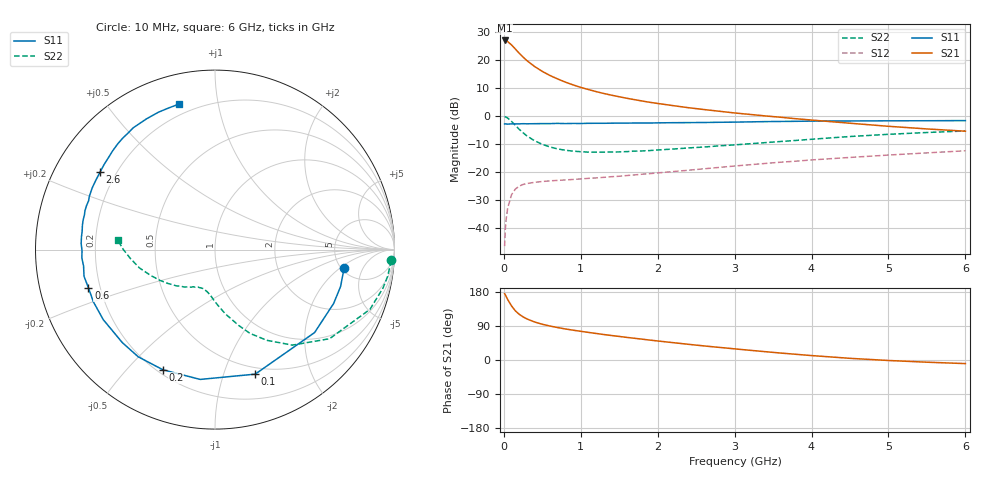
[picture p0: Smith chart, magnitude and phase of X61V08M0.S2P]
! SIEMENS Small Signal Semiconductors
! BFP193W
! Si NPN RF Bipolar Junction Transistor in SOT343
! VCE = 1 V  IC = 8 mA
! Common Emitter S-Parameters:  April 1994
# GHz  S  MA  R  50
!  f  S11  S21  S12  S22
! GHz  MAG  ANG  MAG  ANG  MAG  ANG  MAG  ANG
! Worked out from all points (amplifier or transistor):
!   40 points, 10 MHz to 6 GHz, reference 50 ohm
!   highest |S21| = 27.1 dB at 10 MHz (marker M1)
!   |S21| within 3 dB of that: start of sweep to 147.5 MHz
!   unconditionally stable (mu >= 1): 1.345 GHz to 5.697 GHz
!   at 200 MHz: K = 0.20, MSG = 23.8 dB, |S12| = -25.0 dB
!   at 1.5 GHz: K = 1.06, MAG = 12.8 dB, |S12| = -21.5 dB
!   at 6 GHz: K = 0.98, MSG = 3.5 dB, |S12| = -12.4 dB
!   S11 on the Smith chart (normalised r, x): 10 MHz: 5.32, -2.28; 100 MHz: 0.43, -1.28; 200 MHz: 0.22, -0.63; 600 MHz: 0.15, -0.14; 2.6 GHz: 0.14, +0.30; 6 GHz: 0.14, +0.77
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0.01  0.7269 -8.0  22.77 175.0  0.0047 87.2  0.9836 -3.5
0.02  0.7293 -16.4  22.73 171.6  0.0097 84.2  0.9735 -8.8
0.03  0.726 -24.4  22.54 167.6  0.0142 78.8  0.9602 -12.9
0.05  0.7222 -39.8  21.72 159.5  0.0227 71.9  0.9253 -21.1
0.1  0.7291 -72.1  18.91 142.7  0.0392 56.9  0.8085 -37.9
0.15  0.728 -96.5  15.98 129.7  0.0496 46.4  0.6848 -51.0
0.2  0.7297 -113.4  13.41 120.6  0.056 39.7  0.5825 -60.2
0.25  0.7347 -125.6  11.49 113.8  0.0599 35.0  0.5064 -67.3
0.3  0.7315 -134.9  9.904 108.4  0.0623 31.9  0.4434 -72.6
0.4  0.7348 -147.9  7.77 100.3  0.0654 28.2  0.3631 -80.8
0.5  0.7374 -156.8  6.357 94.3  0.0677 26.7  0.3139 -86.6
0.6  0.7367 -163.2  5.357 89.6  0.0695 25.9  0.2814 -91.4
0.8  0.738 -172.8  4.079 81.9  0.0722 26.6  0.2459 -98.3
1.1  0.7465 177.4  3.009 72.8  0.0771 29.0  0.2272 -106.2
1.3  0.7474 172.0  2.553 67.2  0.0804 31.1  0.2274 -110.3
1.6  0.7527 165.2  2.097 59.6  0.0866 34.1  0.2324 -115.8
2.2  0.7658 153.3  1.549 45.8  0.102 38.6  0.2582 -126.4
2.6  0.7722 146.1  1.318 37.2  0.1143 40.4  0.2805 -133.5
3.2  0.7922 136.1  1.077 25.6  0.1353 41.0  0.3216 -143.9
4.5  0.8223 117.7  0.749 4.4  0.1827 37.5  0.4333 -166.4
5.5  0.8299 108.4  0.592 -5.8  0.2204 32.8  0.511 179.9
6  0.8354 103.9  0.539 -9.5  0.2404 30.4  0.5443 174.5
